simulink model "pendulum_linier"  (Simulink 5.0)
settings: Solver=ode45  StartTime=0.0  StopTime=25  RelTol=1e-6

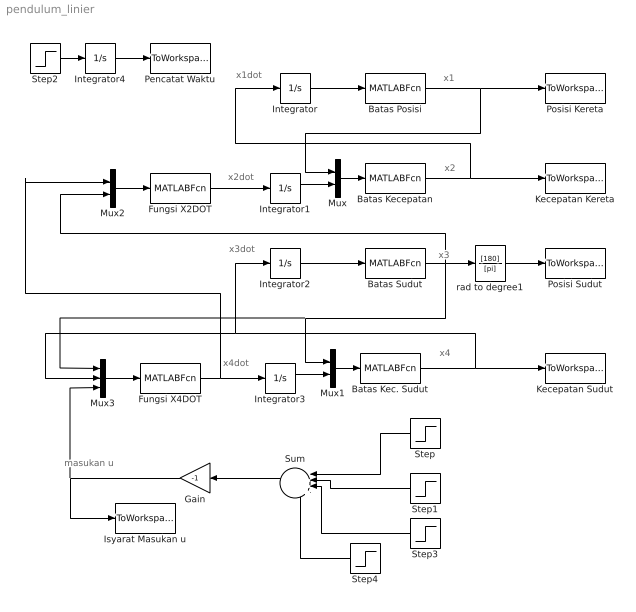
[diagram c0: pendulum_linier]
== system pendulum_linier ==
  note: x1
  note: x2
  note: x3
  note: x4
  note: x1dot
  note: x2dot
  note: x3dot
  note: x4dot
  note: masukan u
  Batas Kec. Sudut : MATLABFcn  MATLABFcn=batas_tetadot
  Batas Kecepatan : MATLABFcn  MATLABFcn=batas_xdot
  Batas Posisi : MATLABFcn  MATLABFcn=batas_x
  Batas Sudut : MATLABFcn  MATLABFcn=batas_teta
  Fungsi X2DOT : MATLABFcn  MATLABFcn=x2dot_lin
  Fungsi X4DOT : MATLABFcn  MATLABFcn=x4dot_lin
  Gain : Gain  Orientation=left  Gain=-1
  Integrator{,1..4} (5 alike) : Integrator
  Isyarat Masukan u : ToWorkspace  VariableName=u  SampleTime=-1  SaveFormat=Array
  Kecepatan Kereta : ToWorkspace  VariableName=kecepatan  SampleTime=-1  SaveFormat=Array
  Kecepatan Sudut : ToWorkspace  VariableName=omega  SampleTime=-1  SaveFormat=Array
  Mux : Mux  Inputs=2
  Mux1 : Mux  Inputs=2
  Mux2 : Mux  Inputs=2
  Mux3 : Mux  Inputs=3
  Pencatat Waktu : ToWorkspace  VariableName=time  SampleTime=-1  SaveFormat=Array
  Posisi Kereta : ToWorkspace  VariableName=posisi  SampleTime=-1  SaveFormat=Array
  Posisi Sudut : ToWorkspace  VariableName=teta  SampleTime=-1  SaveFormat=Array
  Step : Step  Orientation=left  Time=0.1  SampleTime=0
  Step1 : Step  Orientation=left  Time=2  After=-3  SampleTime=0
  Step2 : Step  Time=0  SampleTime=0
  Step3 : Step  Orientation=left  Time=8  After=10  SampleTime=0
  Step4 : Step  Orientation=left  Time=10  After=-8  SampleTime=0  ZeroCross=off
  Sum : Sum  Orientation=left  Inputs=|++++
  rad to degree1 : TransferFcn  Numerator=[180]  Denominator=[pi]
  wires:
  Batas Posisi/1 -> Posisi Kereta/1, Mux/1
  Batas Kecepatan/1 -> Kecepatan Kereta/1, Integrator/1
  Batas Sudut/1 -> rad to degree1/1, Mux1/1, Mux3/1, Mux2/2
  Batas Kec. Sudut/1 -> Kecepatan Sudut/1, Integrator2/1, Mux3/2
  Integrator/1 -> Batas Posisi/1
  Mux/1 -> Batas Kecepatan/1
  Mux1/1 -> Batas Kec. Sudut/1
  rad to degree1/1 -> Posisi Sudut/1
  Integrator2/1 -> Batas Sudut/1
  Integrator3/1 -> Mux1/2
  Integrator1/1 -> Mux/2
  Fungsi X2DOT/1 -> Integrator1/1
  Fungsi X4DOT/1 -> Integrator3/1, Mux2/1
  Mux2/1 -> Fungsi X2DOT/1
  Mux3/1 -> Fungsi X4DOT/1
  Sum/1 -> Gain/1
  Gain/1 -> Mux3/3, Isyarat Masukan u/1
  Step/1 -> Sum/1
  Step1/1 -> Sum/2
  Step2/1 -> Integrator4/1
  Integrator4/1 -> Pencatat Waktu/1
  Step3/1 -> Sum/3
  Step4/1 -> Sum/4
